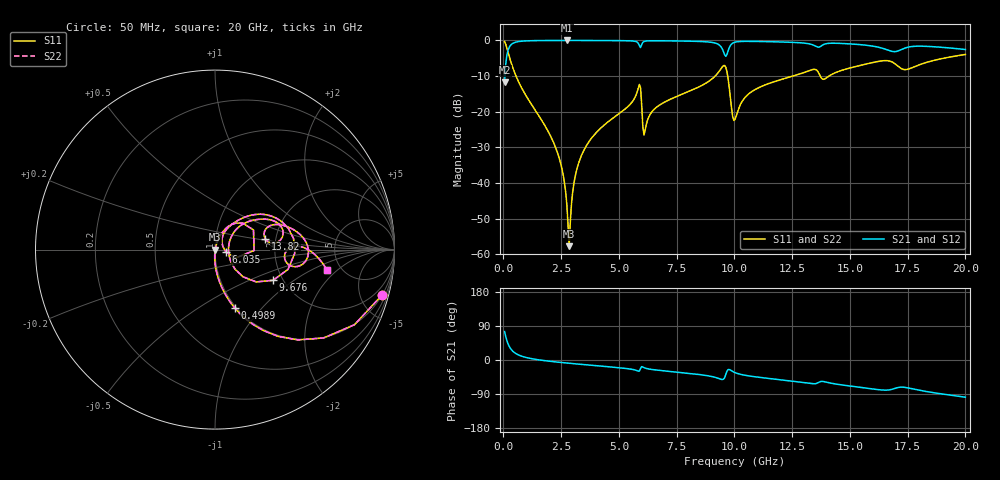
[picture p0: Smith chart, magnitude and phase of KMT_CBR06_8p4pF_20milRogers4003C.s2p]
! Data measured by Modelithics Inc. support@modelithics.com 813-866-6335
! KEMET CBR0603 8.4pF, Pad Width= 0.851mm, Pad Length= 0.64mm, Pad Gap= 0.62mm, 20mil Rogers 4003C substrate Data, January 2022
# hz S ma R 50
! 2 Port Network Data from SP1.SP block
! freq  magS11  angS11  magS21  angS21  magS12  angS12  magS22  angS22
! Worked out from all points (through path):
!   401 points, 50 MHz to 20 GHz, reference 50 ohm
!   highest |S21| = -0.01 dB at 2.743 GHz (marker M1); lowest = -11.8 dB at 50 MHz (marker M2)
!   group delay of S21, straight-line fit = 14.5 ps
!   lowest |S11| = -57.8 dB at 2.843 GHz (marker M3), VSWR 1.00, Z = 50.1 - j0.0155 ohm
!   |S11| at or under -10 dB: 543.7 MHz to 9.167 GHz (8.623 GHz wide, 178 % of centre); 9.708 GHz to 12.53 GHz (2.826 GHz wide, 25.4 % of centre); 13.72 GHz to 14.1 GHz (380.3 MHz wide, 2.73 % of centre)
!   |S22| runs from -57.8 to -0.3 dB; largest |S21 - S12| = 0
!   S11 on the Smith chart (normalised r, x): 50 MHz: 0.98, -7.44; 498.9 MHz: 0.98, -0.72; 6.035 GHz: 1.13, -0.03; 9.676 GHz: 1.78, -0.70; 13.82 GHz: 1.76, +0.23; 20 GHz: 3.86, -1.50
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5e7  0.9663 -15.0  0.2571 74.9  0.2571 74.9  0.9663 -15.0
2.495e8  0.5985 -53.9  0.8002 36.0  0.8002 36.0  0.5985 -53.9
4.98875e8  0.3431 -71.3  0.9384 18.6  0.9384 18.6  0.3431 -71.3
2.2445e9  0.03222 -92.9  0.9982 -4.9  0.9982 -4.9  0.03222 -92.9
2.54375e9  0.01518 -92.2  0.9986 -6.8  0.9986 -6.8  0.01518 -92.2
2.74325e9  0.005013 -83.3  0.9986 -8.0  0.9986 -8.0  0.005013 -83.3
2.843e9  0.001295 -6.9  0.9986 -8.6  0.9986 -8.6  0.001295 -6.9
3.092375e9  0.01176 73.4  0.9985 -10.0  0.9985 -10.0  0.01176 73.4
3.391625e9  0.02487 75.1  0.9982 -11.7  0.9982 -11.7  0.02487 75.1
5.8355e9  0.2137 43.5  0.9156 -29.3  0.9156 -29.3  0.2137 43.5
6.035e9  0.06166 -11.8  0.9385 -18.6  0.9385 -18.6  0.06166 -11.8
6.13475e9  0.05532 45.0  0.9763 -21.4  0.9763 -21.4  0.05532 45.0
6.73325e9  0.1223 60.8  0.9882 -27.3  0.9882 -27.3  0.1223 60.8
9.227e9  0.3318 36.3  0.9043 -46.9  0.9043 -46.9  0.3318 36.3
9.675875e9  0.3662 -27.8  0.6336 -29.6  0.6336 -29.6  0.3662 -27.8
1.0025e10  0.07785 12.9  0.9441 -33.2  0.9441 -33.2  0.07785 12.9
1.0823e10  0.198 43.1  0.9689 -43.7  0.9689 -43.7  0.198 43.1
1.336662e10  0.3881 20.2  0.8725 -62.4  0.8725 -62.4  0.3881 20.2
1.38155e10  0.286 12.3  0.8596 -56.5  0.8596 -56.5  0.286 12.3
1.670825e10  0.514 -5.9  0.7191 -78.8  0.7191 -78.8  0.514 -5.9
1.74065e10  0.3891 -4.6  0.7853 -72.5  0.7853 -72.5  0.3891 -4.6
2e10  0.6354 -10.5  0.7455 -98.2  0.7455 -98.2  0.6354 -10.5
